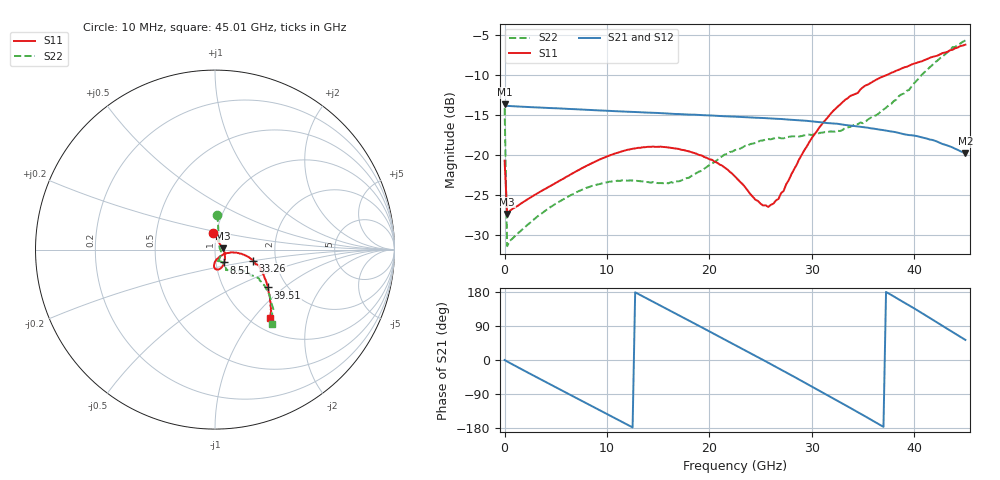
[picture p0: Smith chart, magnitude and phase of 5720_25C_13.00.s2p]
! Device:  ADRF5720
! Description: 0.5dB LSB GaAs MMIC 6-bit Digital Attenuator
! Frequency:  0.000009 -  40 GHz
! Ports:
!	RF1	= Port 1
!	RF2	= Port 2
! Vdd:  3.3 Volt
! Vss:  -3.3 Volt
! Control:  0/3.3 Volt
! State:  13.00 dB attenuation
! Data:  The device was measured using G-S-G Probes on a matrix board.
!  Data was collected using an calibrated 4 port network analyzer.
!  The reference plane for this measurement is at the launchers.
! Note:  Analog Devices supplies this data as a sample of measured data
!  for this product.  Your particular data for this product may vary.
!  Data was taken at 25 degrees C.
!  Analog Devices reserves the right to change this data at anytime.
# GHZ S DB R 45.0
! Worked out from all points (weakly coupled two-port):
!   181 points, 10 MHz to 45.01 GHz, reference 45 ohm
!   highest |S21| = -13.69 dB at 10 MHz (marker M1); lowest = -19.8 dB at 45.01 GHz (marker M2)
!   lowest |S11| = -27.4 dB at 260 MHz (marker M3), VSWR 1.09, Z = 48.9 + j0.794 ohm
!   |S11| at or under -10 dB: start of sweep to 37.31 GHz
!   |S22| runs from -31.4 to -5.7 dB; largest |S21 - S12| = 0.00024
!   S11 on the Smith chart (normalised r, x): 10 MHz: 0.96, +0.18; 8.51 GHz: 1.10, -0.16; 33.26 GHz: 1.52, -0.20; 39.51 GHz: 1.60, -0.78; 45.01 GHz: 1.21, -1.22
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0.01  -20.74 96.5  -13.69 -0.1  -13.69 -0.1  -14.16 86.1
0.26  -27.41 11.0  -13.87 -4.0  -13.88 -4.0  -31.45 16.3
4.26  -24.06 -28.6  -14.13 -61.4  -14.13 -61.3  -26.75 -46.7
7.76  -21.54 -50.1  -14.34 -110.9  -14.34 -110.8  -24.27 -69.3
8.51  -21.06 -54.1  -14.39 -121.5  -14.39 -121.4  -23.91 -72.7
12.01  -19.37 -71.0  -14.60 -170.8  -14.60 -170.8  -23.24 -81.6
15.26  -18.98 -83.2  -14.78 143.1  -14.78 143.1  -23.54 -78.2
16.51  -19.17 -87.1  -14.87 125.3  -14.88 125.4  -23.53 -72.7
19.01  -20.03 -92.0  -15.01 89.8  -15.01 89.8  -22.09 -61.1
21.26  -21.36 -93.3  -15.15 57.6  -15.15 57.6  -20.17 -57.8
22.76  -23.05 -91.0  -15.24 36.1  -15.24 36.1  -19.34 -57.6
24.51  -25.63 -74.6  -15.35 11.0  -15.35 11.0  -18.51 -59.3
25.76  -26.54 -52.0  -15.43 -7.2  -15.43 -7.2  -18.03 -60.4
27.26  -24.53 -22.6  -15.54 -29.3  -15.54 -29.2  -17.94 -60.3
30.26  -17.45 -8.3  -15.84 -73.7  -15.85 -73.7  -17.42 -57.9
33.26  -13.11 -16.1  -16.26 -118.8  -16.26 -118.8  -16.64 -49.7
35.01  -11.53 -21.3  -16.53 -145.3  -16.53 -145.3  -16.04 -45.2
37.76  -9.73 -30.7  -17.08 171.9  -17.08 172.0  -13.64 -35.5
39.51  -8.83 -35.7  -17.53 144.3  -17.53 144.4  -11.87 -34.7
42.01  -7.66 -42.3  -18.23 102.8  -18.23 102.8  -8.42 -38.5
43.76  -6.83 -47.0  -19.08 73.6  -19.08 73.6  -6.50 -46.2
45.01  -6.20 -51.5  -19.83 53.0  -19.83 53.0  -5.67 -52.7
